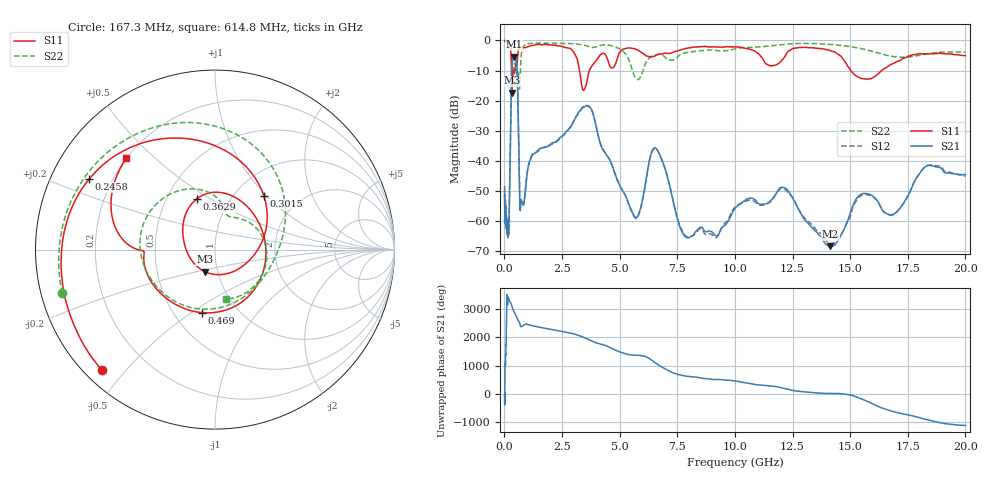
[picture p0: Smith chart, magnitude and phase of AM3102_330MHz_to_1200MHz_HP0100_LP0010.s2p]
! Date/Time: Tue, Sep 11, 2018 5:12 PM
! Network Analyzer: Agilent Technologies E8362B Rev: A.07.50.63
! Sweep from 0.010 to 20.000 GHz, 1601 Points, Sweep Type: LOG
! Power Supply: 4.949 V, 0.001 A
# Hz S DB R 50
!freq MagS11 AngS11 MagS21 AngS21 MagS12 AngS12 MagS22 AngS22
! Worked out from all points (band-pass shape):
!   1601 points, 10 MHz to 20 GHz, reference 50 ohm
!   highest |S21| = -5.35 dB at 416.5 MHz (marker M1); lowest = -68.3 dB at 14.14 GHz (marker M2)
!   |S21| within 3 dB of the highest: 331.8 MHz to 539.6 MHz (207.9 MHz wide, 47.7 % of centre)
!   lowest |S11| = -17.4 dB at 330 MHz (marker M3), VSWR 1.31, Z = 43.3 - j10.8 ohm
!   |S11| at or under -10 dB: 307.9 MHz to 370.3 MHz (62.35 MHz wide, 18.4 % of centre); 3.257 GHz to 3.682 GHz (425.4 MHz wide, 12.3 % of centre); 15.03 GHz to 16.37 GHz (1.345 GHz wide, 8.57 % of centre)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
!   |S22| runs from -16.2 to -0.2 dB; largest |S21 - S12| = 0.008
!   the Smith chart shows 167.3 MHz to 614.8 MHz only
!   S11 on the Smith chart (normalised r, x): 167.3 MHz: 0.05, -0.43; 245.8 MHz: 0.12, +0.26; 301.5 MHz: 1.35, +0.97; 362.9 MHz: 0.70, +0.44; 469 MHz: 0.68, -0.55; 614.8 MHz: 0.20, +0.41
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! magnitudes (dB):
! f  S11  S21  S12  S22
! 10 MHz  0.0  -49.7  -48.5  -0.2
! 35.55 MHz  0.0  -58.6  -59.1  -0.3
! 126.4 MHz  -0.4  -62.5  -64.4  -0.8
! 167.3 MHz  -0.7  -63.1  -64.4  -1.1
! 245.8 MHz  -1.9  -41.3  -41.5  -2.0
! 301.5 MHz  -7.8  -16.1  -16.2  -4.8
! 330 MHz  -17.4  -8.6  -8.6  -8.8
! 362.9 MHz  -10.4  -6.1  -6.2  -10.1
! 416.5 MHz  -11.0  -5.3  -5.4  -8.0
! 447.2 MHz  -9.7  -5.5  -5.6  -7.5
! 469 MHz  -8.9  -5.8  -5.8  -7.6
! 551.2 MHz  -7.5  -9.8  -9.9  -13.9
! 614.8 MHz  -3.0  -31.3  -31.3  -11.0
! 689.1 MHz  -2.3  -56.5  -56.0  -11.3
! 1.59 GHz  -1.4  -35.7  -35.8  -0.9
! 3.651 GHz  -10.7  -22.0  -21.7  -2.0
! 5.652 GHz  -2.8  -58.5  -58.9  -12.1
! 6.58 GHz  -4.9  -35.8  -36.1  -4.8
! 7.882 GHz  -2.7  -65.3  -65.1  -4.0
! 12.09 GHz  -6.1  -48.8  -49.1  -1.3
! 14.14 GHz  -3.4  -68.3  -67.5  -1.3
! 20 GHz  -5.0  -44.5  -45.1  -3.8
